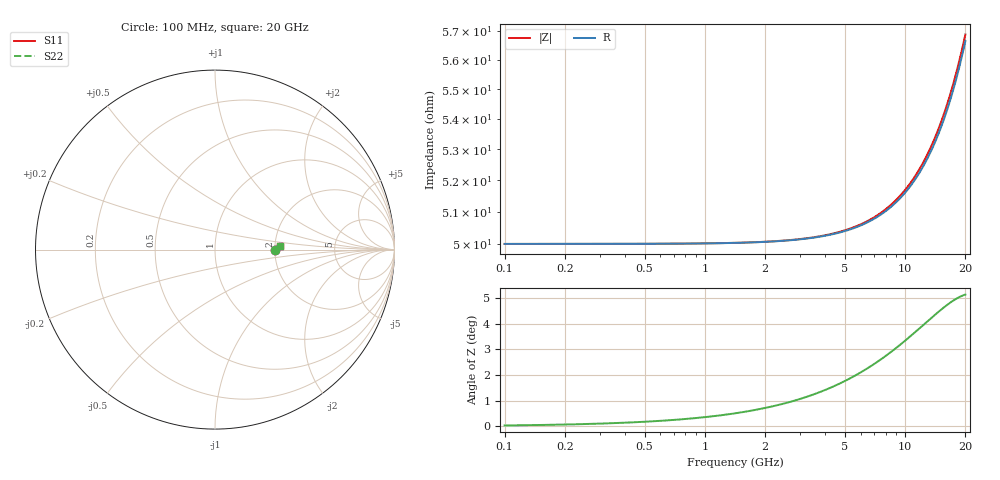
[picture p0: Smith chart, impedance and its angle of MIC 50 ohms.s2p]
! Vishay ElectroFilms Inc.
! MIC001 5000B - 50 Ohm in Series Configuration
! March 2012
# GHz S MA R 50
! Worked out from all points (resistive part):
!   233 points, 100 MHz to 20 GHz, reference 50 ohm
!   read as one part in series: R = 50 ohm at 102.3 MHz
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0.1  0.3333 0.0  0.6667 -0.0  0.6667 -0.0  0.3333 0.0
0.2436751  0.3333 0.1  0.6667 -0.0  0.6667 -0.0  0.3333 0.1
0.5937753  0.3334 0.1  0.6666 -0.1  0.6666 -0.1  0.3334 0.1
0.9375335  0.3334 0.2  0.6666 -0.1  0.6666 -0.1  0.3334 0.2
1.414214  0.3335 0.3  0.6665 -0.2  0.6665 -0.2  0.3335 0.3
2.284535  0.3337 0.5  0.6663 -0.3  0.6663 -0.3  0.3337 0.5
3.446086  0.3342 0.8  0.6658 -0.4  0.6658 -0.4  0.3342 0.8
4.532574  0.3349 1.1  0.6652 -0.5  0.6652 -0.5  0.3349 1.1
5.695439  0.3358 1.3  0.6643 -0.7  0.6643 -0.7  0.3358 1.3
6.995058  0.337 1.6  0.6632 -0.8  0.6632 -0.8  0.337 1.6
8.397251  0.3387 1.9  0.6616 -1.0  0.6616 -1.0  0.3387 1.9
9.630449  0.3403 2.1  0.66 -1.1  0.66 -1.1  0.3403 2.1
10.79537  0.3421 2.3  0.6583 -1.2  0.6583 -1.2  0.3421 2.3
12.10121  0.3444 2.6  0.6562 -1.3  0.6562 -1.3  0.3444 2.6
13.56501  0.3471 2.8  0.6535 -1.5  0.6535 -1.5  0.3471 2.8
14.52696  0.3491 2.9  0.6515 -1.5  0.6515 -1.5  0.3491 2.9
15.20587  0.3506 3.0  0.6501 -1.6  0.6501 -1.6  0.3506 3.0
16.66035  0.354 3.1  0.6468 -1.7  0.6468 -1.7  0.354 3.1
17.43896  0.356 3.2  0.6449 -1.7  0.6449 -1.7  0.356 3.2
18.25396  0.3581 3.2  0.6428 -1.8  0.6428 -1.8  0.3581 3.2
19.10705  0.3604 3.3  0.6405 -1.8  0.6405 -1.8  0.3604 3.3
20  0.3629 3.3  0.638 -1.9  0.638 -1.9  0.3629 3.3
